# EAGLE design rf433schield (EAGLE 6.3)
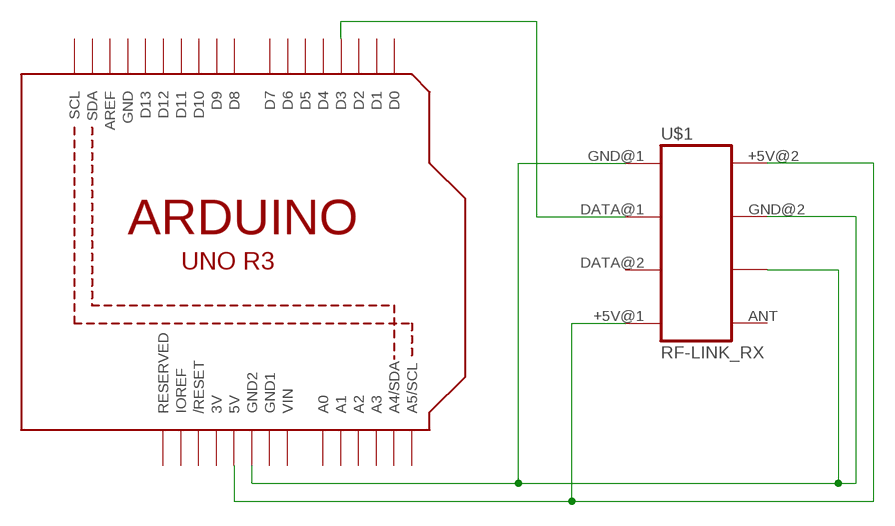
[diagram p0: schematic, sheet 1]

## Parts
U1  ARDUINOR3-DIMENSION  [ARDUINOR3]
U$1  RF-LINK_RX  [RF-LINK_RX]

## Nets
N$1: U1.D3 U$1.DATA@1(DATA_OUT)
N$2: U1.5V U$1.+5V@1(VCC1) U$1.+5V@2(VCC2)
N$3: U1.GND2 U$1.GND@1(GND1) U$1.GND@2(GND2) U$1.GND@3(GND3)
Unconnected: U1.A0 U1.A1 U1.A2 U1.A3 U1.A4(A4/SDA) U1.A5(A5/SCL) U1.AREF U1.D0 U1.D1 U1.D2 U1.D4 U1.D5 U1.D6 U1.D7 U1.D8 U1.D9 U1.D10 U1.D11 U1.D12 U1.D13 U1.IOREF U1.RESERVED U1.RESET(/RESET) U1.SCL U1.SDA U$1.ANT U$1.DATA@2(LINEAR_OUT)

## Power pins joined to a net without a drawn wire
3V: U1.3V
GND: U1.GND
GND1: U1.GND1
VIN: U1.VIN

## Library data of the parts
U1 = adafruit:ARDUINOR3: This is a new object for the new Arduino R3 - with extra pins that you may want to use (such as IOref, and duplicated A4/A5
U$1 = RFM:RF-LINK_RX: RF Link receivers- WRL-8947, 8948, 8949, 8950

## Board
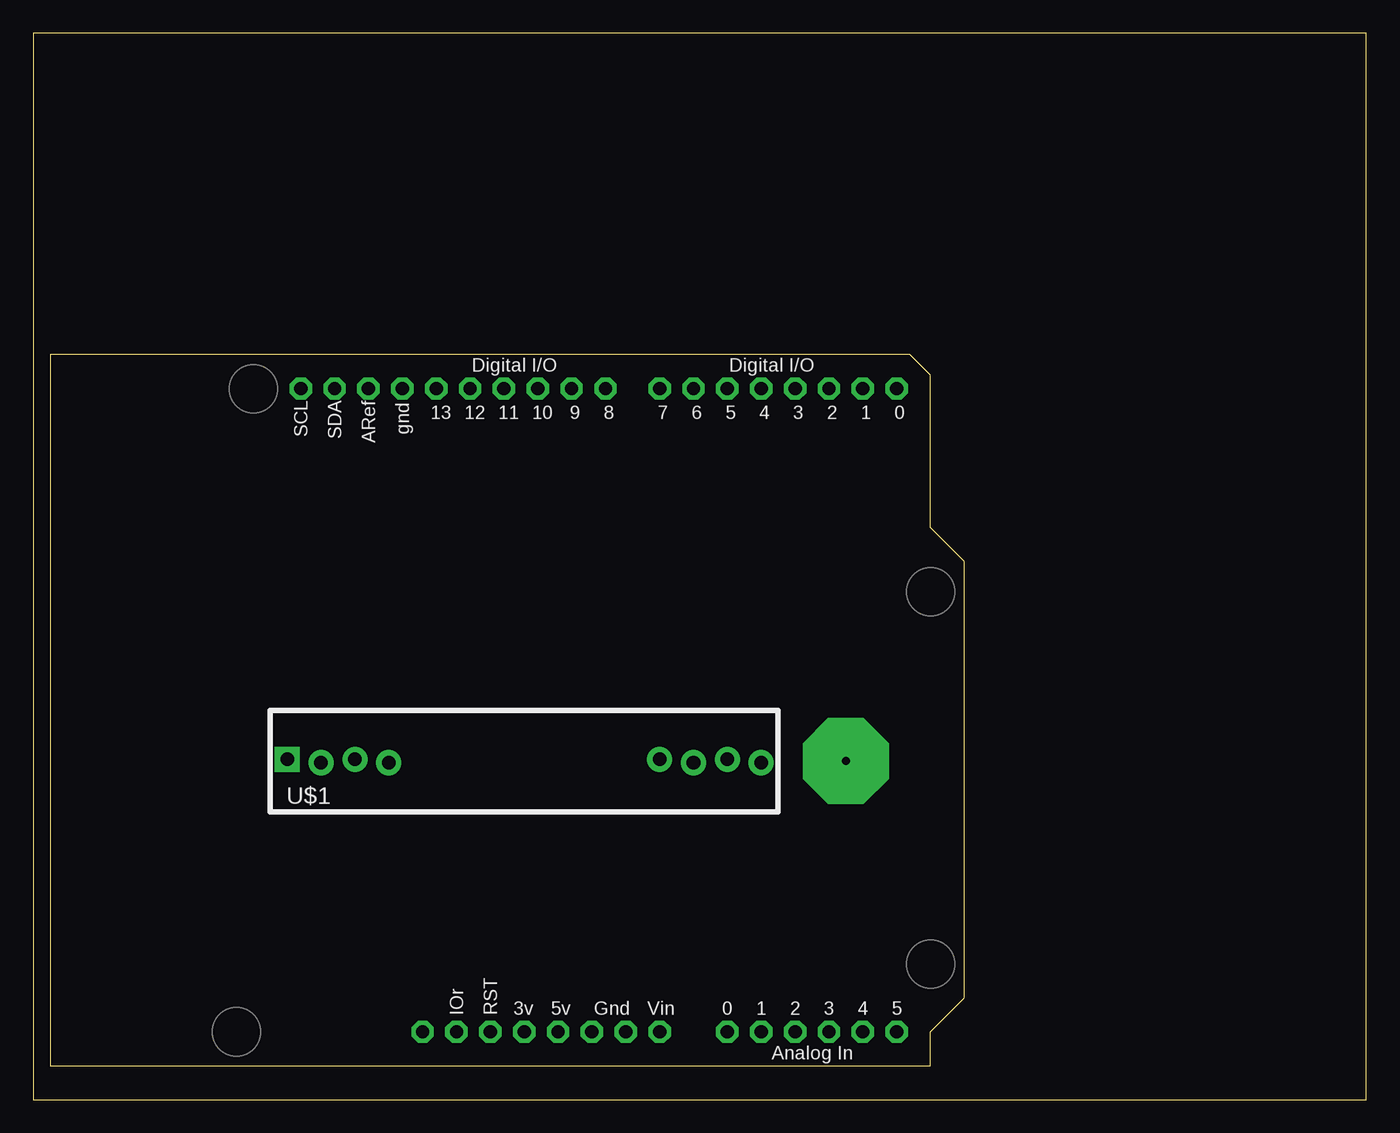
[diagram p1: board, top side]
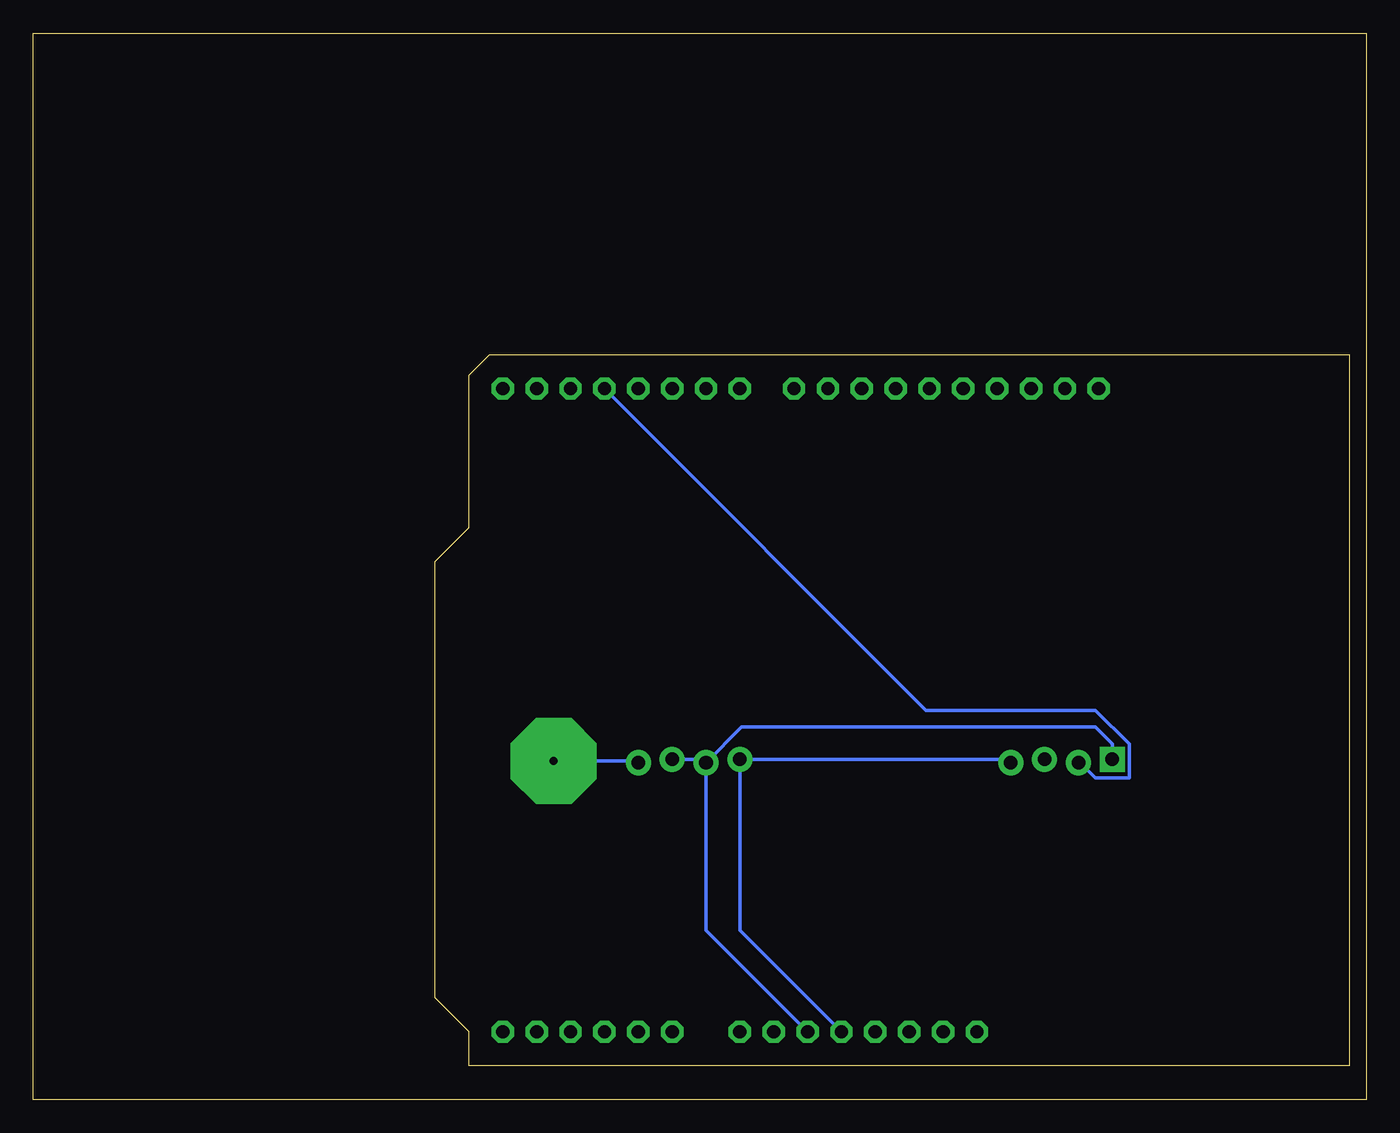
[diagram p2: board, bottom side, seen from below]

Size 100 x 80 mm. Coordinates in mm from the lower left corner, seen from the top.
Outline: 0,0 100,0 100,80 0,80 0,0
Copper layers (1*16): Top 0.035mm / dielectric 1.5mm / Bottom 0.035mm
Design rules "default": minimum track width 10mil, minimum drill 24mil, track to track 8mil, track to pad 8mil, pad to pad 8mil, via to via 8mil, smd to smd 8mil, copper to edge 40mil, drill to drill 8mil, minimum pad ring 10mil, minimum via ring 8mil, stop-mask expansion 4mil, vias tented up to drill 0mil, thermal gap 10mil

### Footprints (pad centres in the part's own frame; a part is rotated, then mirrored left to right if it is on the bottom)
ARDUINOR3 = drill 1 pad 1.676 octagon: 3V 35.56,2.54; 5V 38.1,2.54; A0 50.8,2.54; A1 53.34,2.54; A2 55.88,2.54; A3 58.42,2.54; A4 60.96,2.54; A5 63.5,2.54; AREF 23.876,50.8; D0 63.5,50.8; D1 60.96,50.8; D2 58.42,50.8; D3 55.88,50.8; D4 53.34,50.8; D5 50.8,50.8; D6 48.26,50.8; D7 45.72,50.8; D8 41.656,50.8; D9 39.116,50.8; D10 36.576,50.8; D11 34.036,50.8; D12 31.496,50.8; D13 28.956,50.8; GND 26.416,50.8; GND1 43.18,2.54; GND2 40.64,2.54; IOREF 30.48,2.54; RESERVED 27.94,2.54; RESET 33.02,2.54; SCL 18.796,50.8; SDA 21.336,50.8; VIN 45.72,2.54
RF-LINK_RX = drill 1.016 pad 1.88: +5V@1 7.62,-0.127; +5V@2 27.94,0.127; ANT 35.56,-0.127; DATA@1 2.54,-0.127; DATA@2 5.08,0.127; GND@2 30.48,-0.127; GND@3 33.02,0.127 | drill 1.016 pad 1.88 square: GND@1 0,0.127

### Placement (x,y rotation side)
U1  1.27,2.54 0 top
U$1  19.05,25.4 0 top

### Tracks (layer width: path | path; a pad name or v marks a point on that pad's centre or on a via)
N$1
  Bottom 0.254: U1.D3 33.02,29.21 20.32,29.21 17.78,26.67 17.78,24.13 20.32,24.13 21.59,25.4 U$1.DATA@1
N$2
  Bottom 0.254: U$1.+5V@1 26.92,25.53 U$1.+5V@2 46.99,12.7 U1.5V
N$3
  Bottom 0.254: U$1.GND@1 19.05,26.67 20.32,27.94 46.86,27.94 U$1.GND@2 | U1.GND2 49.53,12.7 U$1.GND@2 | U$1.GND@3 49.78,25.53 U$1.GND@2
N$4  (via drill 0.6 pad 6.45)
  other vias: 60.96,25.4
N$6
  Bottom 0.254: 54.61,25.4 59.69,25.4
